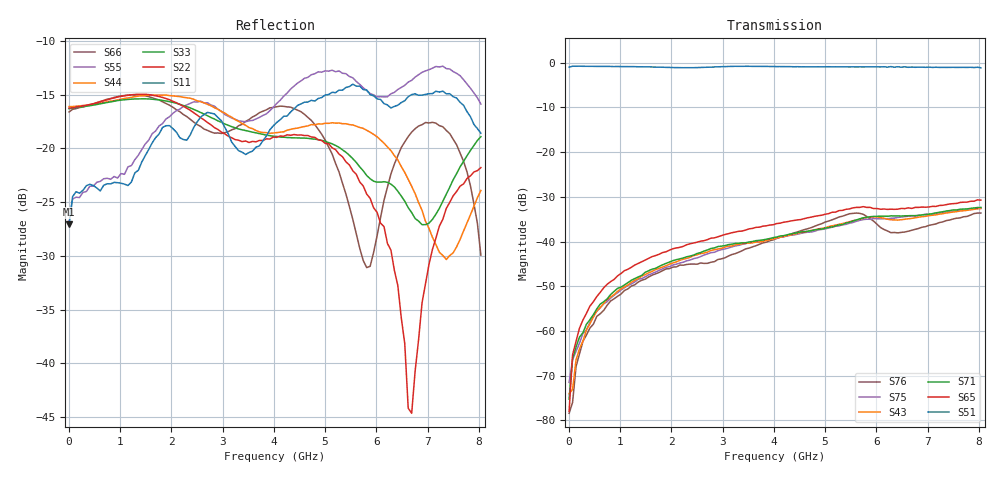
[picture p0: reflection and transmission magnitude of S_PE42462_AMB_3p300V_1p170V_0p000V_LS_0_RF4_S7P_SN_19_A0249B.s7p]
! Device ID: PE42462
! File Path: z:\PE42462\DataSheet S-parameter-6T\AMB\3p300\LS_0_RF4\PE42462_AMB_3p300V_1p170V_0p000V_LS_0_RF4_S7P_SN_19_A0249B.s7p
! Serial: 19
! Lot: A0249B
! Temp: AMB
! VDD: 3.300
! VSS: 0.000
! Control_Hi: 1.170
! Control_Lo: 0.000
! Logic State: LS_0_RF4
! Port 1:
! Port 2:
! Port 3:
! Port 4:
! Port 5:
! Port 6:
! Port 7:
! ThroughPath:1-5
! IDD: 0.0001069816
! ISS/IDD2: 1.43e-008
! IDMM3/IDD3: -2.661e-007
! Comment:
#  Hz  S  RI  R  50
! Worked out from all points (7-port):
!   120 points, 10 MHz to 8.037 GHz, reference 50 ohm
!   strongest paths, dB at 10 MHz, 2.034 GHz, 4.057 GHz, 6.08 GHz, 8.037 GHz:
!     S51: -1.0, -1.1, -0.9, -1.0, -1.1
!     S65: -78.0, -41.6, -36.0, -32.8, -30.7
!     S71: -75.3, -44.3, -39.0, -34.3, -32.4
!     S43: -74.0, -44.8, -39.2, -34.6, -32.6
!     S75: -71.5, -45.3, -39.3, -34.9, -32.4
!     S76: -78.4, -45.7, -39.3, -36.9, -33.6
!   lowest |S11| = -27.1 dB at 10 MHz (marker M1), VSWR 1.09, Z = 53.2 - j3.24 ohm
!   |S11| at or under -10 dB: start of sweep to end of sweep
